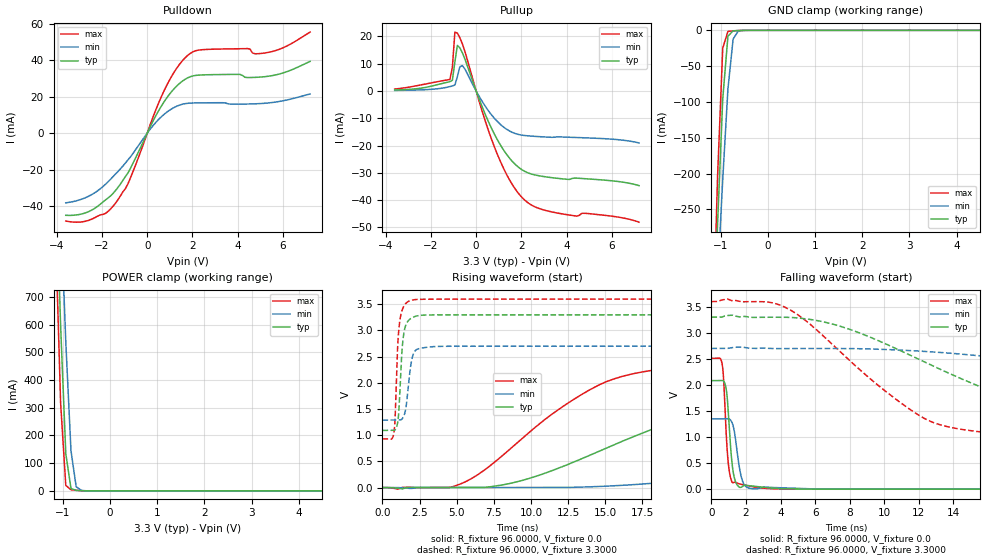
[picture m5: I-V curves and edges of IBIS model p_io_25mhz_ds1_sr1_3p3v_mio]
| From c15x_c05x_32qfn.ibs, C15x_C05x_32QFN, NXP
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[Model] p_io_25mhz_ds1_sr1_3p3v_mio
|   Model p_io_25mhz_ds1_sr1_3p3v_mio
| This model was characterised for following simulation conditions:
| External (pad) voltage:
|   - Typ: 3.3V,   - Min: 2.7V,   - Max: 3.6V
| Library cells for typ/min/max conditions are connected as defined below:
|  pad - External Pad
|  ipp_do_lv - Core Input
|  ipp_obe_lv - Output Buffer Enable
|  IOGC - NC
|  REFH3V3 - REFH3V3
|  REFL3V3 - REFL3V3
|  ZI - NC
|  abut_ncal_vddio[1] - vddio
|  abut_ncal_vddio[2] - vddio
|  abut_ncal_vddio[3] - vssio
|  abut_ncal_vddio[4] - vddio
|  abut_ncal_vddio[5] - vddio
|  abut_ncal_vddio[6] - vssio
|  abut_pcal_vddio[1] - vssio
|  abut_pcal_vddio[2] - vssio
|  abut_pcal_vddio[3] - vddio
|  abut_pcal_vddio[4] - vssio
|  abut_pcal_vddio[5] - vssio
|  abut_pcal_vddio[6] - vddio
|  ipp_do_1p8v - ipp_do_1p8v
|  ipp_dse_lv - vdd_lv
|  ipp_eftd_lv - NC
|  ipp_ina_mux_vddio - NC
|  ipp_ina_mux_vddio[0] - NC
|  ipp_ina_mux_vddio[1] - NC
|  ipp_ina_r0_vddio - NC
|  ipp_ina_r0a_vddio - NC
|  ipp_ina_r0b_vddio - NC
|  ipp_ina_r0c_vddio - NC
|  ipp_ina_r0d_vddio - NC
|  ipp_ina_r0e_vddio - NC
|  ipp_ina_r0f_vddio - NC
|  ipp_ina_r300_vddio - NC
|  ipp_ina_r300a_vddio - NC
|  ipp_ina_r300b_vddio - NC
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Model_type I/O
Polarity   Non-Inverting
Enable   Active-High
Vinl =   0.9900V
Vinh =   2.3100V
Vmeas =  1.6500V
Cref =   30.0000pF
Rref =   1.0000M
Vref =   3.3000V
C_comp   1.2813pF   1.2310pF   1.3501pF
|C_comp_pullup   0.5366pF   0.5680pF   0.5153pF
|C_comp_pulldown   0.6536pF   0.6897pF   0.6249pF
[Model Spec]
| variable   typ   min   max
Vinh   2.3100V   1.8900V   2.5200V
Vinl   0.9900V   0.8100V   1.0800V
[Temperature Range]   25.0000   0.1250k   -40.0000
[Voltage Range]   3.3000V   2.7000V   3.6000V
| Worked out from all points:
|   slope of the pulldown table from 0 to 0.495 V, typ, clamps not added: 40.9 ohm
|   slope of the pullup table from 0 to 0.495 V, typ, clamps not added: 47.8 ohm
|   GND clamp passes 1 mA (typ) near -0.74 V on its own axis
|   POWER clamp passes 1 mA (typ) near -0.62 V on its own axis
|   rising waveform, R_fixture 96.0000, V_fixture 0.0: 20-80 % time 12.3ns typ, 26.1ns min, 7.34ns max; typ from 0 V to 2.08 V
|   rising waveform, R_fixture 96.0000, V_fixture 3.3000: 20-80 % time 276ps typ, 352ps min, 249ps max; typ from 1.09 V to 3.3 V
|   falling waveform, R_fixture 96.0000, V_fixture 0.0: 20-80 % time 285ps typ, 363ps min, 251ps max; typ from 2.08 V to 0 V
|   falling waveform, R_fixture 96.0000, V_fixture 3.3000: 20-80 % time 9.46ns typ, 20.5ns min, 5.74ns max; typ from 3.3 V to 1.09 V
[Pulldown]
|Voltage   I(typ)   I(min)   I(max)
-3.6V     -44.98mA   -38.16mA   -48.14mA
-2.5V     -42.45mA   -33.96mA   -47.35mA
-1.84V    -36.56mA   -27.93mA   -43.93mA
-1.4V     -31.43mA   -22.35mA   -38.33mA
-850mV    -21.79mA   -14.63mA   -27.72mA
800mV     18.2mA     10.89mA    24.65mA
1.35V     26.4mA     15.02mA    36.44mA
1.9V      30.96mA    16.49mA    43.72mA
4.43V     30.51mA    16mA       46.38mA
4.76V     30.6mA     16.11mA    43.52mA
5.31V     31.15mA    16.54mA    44.2mA
7.2V      39.37mA    21.51mA    55.42mA
[Pullup]
|Voltage   I(typ)   I(min)   I(max)
-3.6V     375.6uA    207.2uA    723.4uA
-1.16V    3.421mA    1.609mA    4.222mA
-1.05V    3.932mA    1.826mA    8.69mA
-940mV    10.66mA    2.21mA     21.59mA
-830mV    16.71mA    5.23mA     21.25mA
-720mV    15.83mA    8.864mA    19.49mA
-610mV    14.01mA    9.303mA    17.31mA
820mV     -16.02mA   -10.13mA   -20.77mA
1.48V     -24.67mA   -14.68mA   -32.64mA
2.03V     -28.89mA   -16.19mA   -39.05mA
3.35V     -31.77mA   -16.98mA   -44.33mA
7.2V      -34.69mA   -19.05mA   -48.09mA
[GND_clamp]
|Voltage   I(typ)   I(min)   I(max)
-3.6V     -5.285A    -4.099A    -6.854A
-1.18V    -466mA     -495.3mA   -458.9mA
-1.07V    -271.1mA   -348.5mA   -204.6mA
-960mV    -95.66mA   -207.9mA   -24.82mA
-850mV    -8.126mA   -81.84mA   -1.536mA
-740mV    -740.4uA   -12.14mA   -755uA
-630mV    -283.6uA   -928.1uA   -319.7uA
-300mV    -497.8nA   -2.865uA   -109.5nA
7.2V      0A         0A         0A
[POWER_clamp]
|Voltage   I(typ)   I(min)   I(max)
-3.6V     14.48A     12.95A     16.35A
-1.16V    1.177A     1.535A     951.2mA
-1.05V    598.3mA    1.032A     318mA
-940mV    134.2mA    537.3mA    19.98mA
-830mV    8.694mA    145.4mA    4.231mA
-720mV    2.123mA    15.37mA    2.22mA
-610mV    848.6uA    1.85mA     839.5uA
7.2V      0A         0A         0A
[Ramp]
| variable   typ   min   max
dV/dt_r  1.2494/12.3178n   0.8019/26.1429n   1.5064/7.3439n
dV/dt_f  1.3247/9.4639n   0.8433/20.5314n   1.6022/5.7376n
R_load = 96.0000
[Rising Waveform]
R_fixture= 96.0000
V_fixture= 0.0
V_fixture_min= 0.0
V_fixture_max= 0.0
|time   V(typ)   V(min)   V(max)
0s        3.132nV    106.7nV    10.54nV
4.808ns   -80.06uV   -247.9uV   23.94mV
8.95ns    102.4mV    14.08uV    825.8mV
11.95ns   381.4mV    644.8uV    1.51V
15.13ns   760mV      27.05mV    2.028V
21.76ns   1.468V     177.7mV    2.347V
32.28ns   1.89V      547.2mV    2.459V
43.95ns   2.004V     934.8mV    2.494V
55.32ns   2.046V     1.13V      2.504V
127.4ns   2.082V     1.337V     2.511V
[Rising Waveform]
R_fixture= 96.0000
V_fixture= 3.3000
V_fixture_min= 2.7000
V_fixture_max= 3.6000
|time   V(typ)   V(min)   V(max)
0s        1.092V     1.289V     929.6mV
776ps     1.091V     1.289V     1.053V
851.9ps   1.103V     1.289V     1.345V
1.067ns   1.334V     1.289V     2.901V
1.264ns   2.387V     1.298V     3.333V
1.383ns   2.832V     1.337V     3.434V
1.548ns   3.084V     1.472V     3.509V
1.945ns   3.236V     2.402V     3.578V
2.287ns   3.276V     2.634V     3.592V
127.4ns   3.3V       2.7V       3.6V
[Falling Waveform]
R_fixture= 96.0000
V_fixture= 0.0
V_fixture_min= 0.0
V_fixture_max= 0.0
|time   V(typ)   V(min)   V(max)
0s        2.083V     1.349V     2.511V
634.5ps   2.086V     1.348V     2.371V
717.6ps   2.069V     1.348V     2.041V
889.1ps   1.84V      1.35V      866mV
1.009ns   1.306V     1.348V     402.3mV
1.167ns   579.9mV    1.295V     153.1mV
1.429ns   117.1mV    873.1mV    123.5mV
1.881ns   71.9mV     95.8mV     81.09mV
3.284ns   27.42mV    36mV       12.14mV
127.4ns   228.8nV    4.573uV    22.67nV
[Falling Waveform]
R_fixture= 96.0000
V_fixture= 3.3000
V_fixture_min= 2.7000
V_fixture_max= 3.6000
|time   V(typ)   V(min)   V(max)
0s        3.3V       2.7V       3.6V
4.228ns   3.298V     2.698V     3.496V
7.486ns   3.123V     2.699V     2.626V
12.29ns   2.447V     2.644V     1.364V
17.44ns   1.717V     2.492V     1.048V
20.53ns   1.424V     2.363V     999.4mV
24.94ns   1.274V     2.159V     966mV
35.93ns   1.154V     1.677V     939.2mV
46.3ns    1.119V     1.478V     932.9mV
127.4ns   1.092V     1.294V     929.6mV
